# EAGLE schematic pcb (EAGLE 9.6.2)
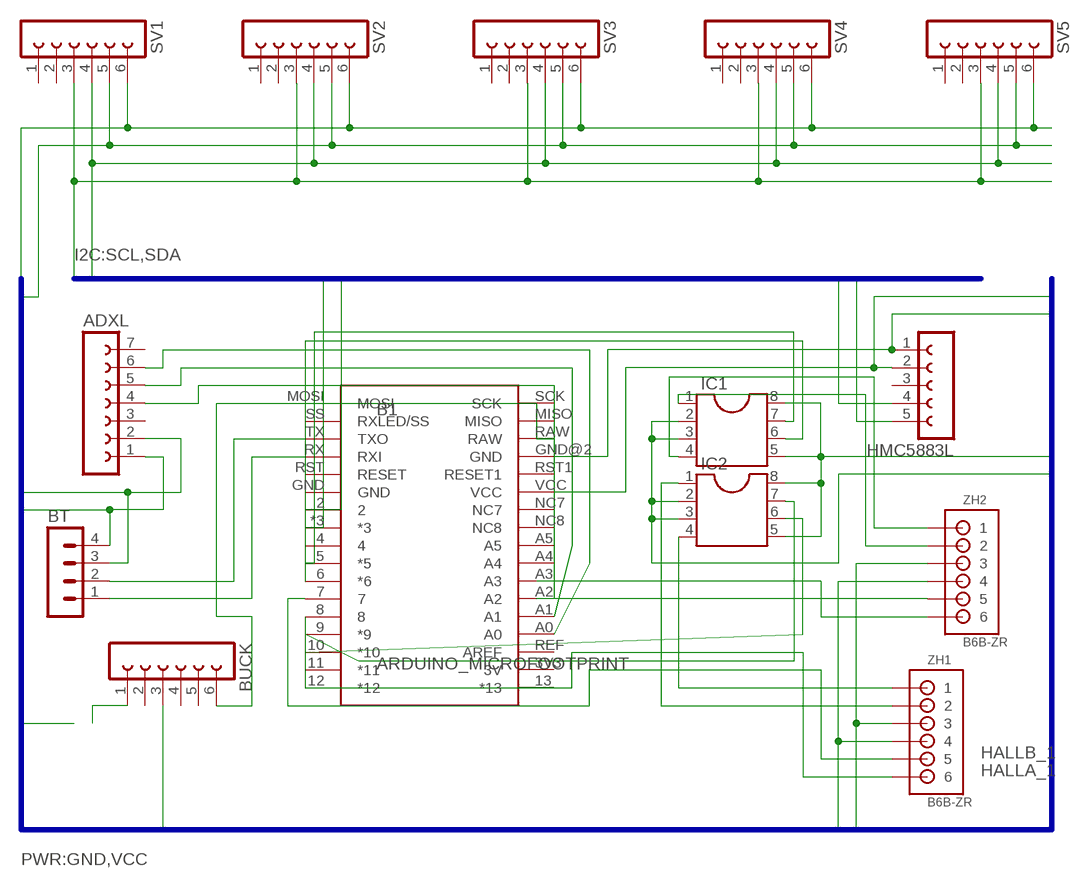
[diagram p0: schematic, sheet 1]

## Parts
ADXL  FE07-1  [FE07]
B1  ARDUINO_MICROFOOTPRINT  [ARDUINO-MICRO]
BT  MA04-1  [MA04-1]
BUCK  FE06-1  [FE06]
HMC5883L  FE05-1  [FE05-1]
IC1  DIL8S  [SOCKET-08]
IC2  DIL8S  [SOCKET-08]
SV1  FE06-1  [FE06]
SV2  FE06-1  [FE06]
SV3  FE06-1  [FE06]
SV4  FE06-1  [FE06]
SV5  FE06-1  [FE06]
ZH1  B6B-ZR  [B6B-ZR]
ZH2  B6B-ZR  [B6B-ZR]

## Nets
GND: ADXL.2 B1.GND@2(GND) BT.3 BUCK.3 HMC5883L.1 IC1.5 IC1.8 IC2.5 IC2.8 SV1.5 SV2.5 SV3.5 SV4.5 SV5.5 ZH1.4 ZH2.4
HALLA_1: B1.8 ZH1.6
HALLB_1: B1.7 ZH1.5
N$1: B1.9(*9) IC2.7
N$2: B1.TX(TXO) BT.2
N$3: B1.10(*10) IC2.6
N$4: ADXL.4 B1.A2
N$5: ADXL.5 B1.A1
N$6: ADXL.6 B1.A0
N$7: BUCK.1
N$8: B1.RAW BUCK.6
N$9: B1.5(*5) IC1.7
N$10: B1.6(*6) IC1.6
N$11: ZH2.5
N$12: ZH2.6
N$13: IC1.1 ZH2.2
N$14: IC1.4 ZH2.1
N$15: IC2.4 ZH1.1
N$16: IC2.1 ZH1.2
RX: B1.RX(RXI) BT.1
SCL: B1.*3 HMC5883L.4 SV1.4 SV2.4 SV3.4 SV4.4 SV5.4
SDA: B1.2 HMC5883L.5 SV1.3 SV2.3 SV3.3 SV4.3 SV5.3
VCC: ADXL.1 B1.VCC BT.4 HMC5883L.2 IC1.2 IC1.3 IC2.2 IC2.3 SV1.6 SV2.6 SV3.6 SV4.6 SV5.6 ZH1.3 ZH2.3
Unconnected: ADXL.3 ADXL.7 B1.3V3(3V) B1.4 B1.11(*11) B1.12(*12) B1.13(*13) B1.A3 B1.A4 B1.A5 B1.GND B1.MISO B1.MOSI B1.NC7 B1.NC8 B1.REF(AREF) B1.RST1(RESET1) B1.RST(RESET) B1.SCK B1.SS(RXLED/SS) BUCK.2 BUCK.4 BUCK.5 HMC5883L.3 SV1.1 SV1.2 SV2.1 SV2.2 SV3.1 SV3.2 SV4.1 SV4.2 SV5.1 SV5.2

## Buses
I2C:SCL,SDA
PWR:GND,VCC

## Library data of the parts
ADXL = con-lsta:FE07-1: FEMALE HEADER; OC_FARNELL: unknown; OC_NEWARK: unknown
B1 = Arduino Micro1:ARDUINO_MICRO
BT = con-lstb:MA04-1: PIN HEADER; OC_FARNELL: unknown; OC_NEWARK: unknown
BUCK SV1-SV5 = con-lsta:FE06-1: FEMALE HEADER; OC_FARNELL: unknown; OC_NEWARK: unknown
HMC5883L = con-lsta:FE05-1: FEMALE HEADER; OC_FARNELL: unknown; OC_NEWARK: unknown
IC1 IC2 = ic-package:DIL8: Dual In Line / Socket
ZH1 ZH2 = JST ZH:B6B-ZR: JST-ZH Connector 6 pol, 1.5mm pitch Package: B6B-ZR Source: http://www.jst-mfg.com/product/pdf/eng/eZH.pdf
